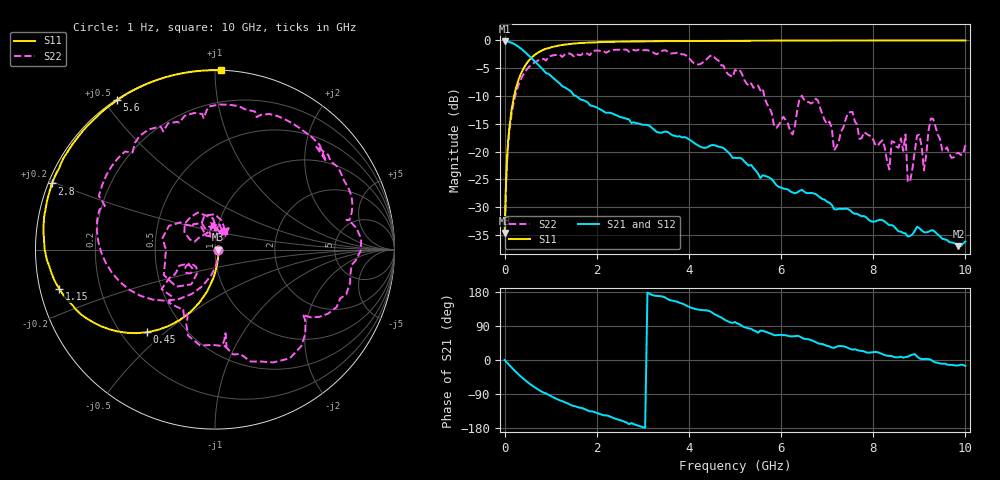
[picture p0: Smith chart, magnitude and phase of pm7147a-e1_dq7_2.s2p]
# GHz S DB R 50
! S-Parameters data
! Freq  dbS11  angS11  dbS21  angS21  dbS12  angS12  dbS22  angS22
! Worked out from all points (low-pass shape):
!   279 points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, 1 Hz to 10 GHz, reference 50 ohm
!   highest |S21| = -0.16 dB at 158.5 Hz (marker M1); lowest = -37.0 dB at 9.85 GHz (marker M2)
!   |S21| within 3 dB of the highest: start of sweep to 580.1 MHz
!   lowest |S11| = -34.6 dB at 100 Hz (marker M3), VSWR 1.04, Z = 51.9 - j1.4e-05 ohm
!   |S11| at or under -10 dB: start of sweep to 206.4 MHz
!   |S22| runs from -34.6 to -1.6 dB; largest |S21 - S12| = 0
!   S11 on the Smith chart (normalised r, x): 1 Hz: 1.04, -0.00; 450 MHz: 0.30, -0.44; 1.15 GHz: 0.06, -0.12; 2.8 GHz: 0.01, +0.20; 5.6 GHz: 0.00, +0.54; 10 GHz: 0.00, +1.03
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1e-09  -34.62 -0.0  -0.16 -0.0  -0.16 -0.0  -34.62 -0.0
1e-07  -34.62 -0.0  -0.16 -0.0  -0.16 -0.0  -34.62 -0.0
1.585e-07  -34.62 -0.0  -0.16 -0.0  -0.16 -0.0  -34.62 -0.0
0.15  -12.55 -100.5  -0.42 -19.5  -0.42 -19.5  -13.35 -108.9
0.45  -4.48 -129.5  -2.14 -53.9  -2.14 -53.9  -5.57 -154.8
1.15  -0.96 -165.9  -7.41 -103.8  -7.41 -103.8  -2.58 136.9
1.7  -0.44 178.6  -10.73 -127.8  -10.73 -127.8  -2.33 102.7
2.8  -0.18 157.9  -14.72 -169.0  -14.72 -169.0  -1.70 39.9
3.35  -0.13 149.9  -16.57 168.8  -16.57 168.8  -2.21 11.1
4.55  -0.09 134.6  -18.84 121.5  -18.84 121.5  -3.01 -62.8
5.05  -0.06 129.0  -21.14 96.3  -21.14 96.3  -5.50 -91.7
5.6  -0.05 123.2  -24.26 77.1  -24.26 77.1  -8.63 -143.5
6.25  -0.02 116.7  -27.34 62.5  -27.34 62.5  -16.93 -136.8
6.7  -0.02 112.6  -27.50 50.2  -27.50 50.2  -11.08 176.8
8.35  -0.01 99.1  -33.25 10.6  -33.25 10.6  -23.22 99.3
8.7  -0.00 96.6  -34.72 7.8  -34.72 7.8  -16.91 57.4
8.8  -0.00 95.9  -35.17 11.9  -35.17 11.9  -25.33 85.1
9  -0.00 94.5  -33.77 4.5  -33.77 4.5  -16.95 79.6
9.1  -0.00 93.9  -34.48 2.4  -34.48 2.4  -23.36 84.6
9.25  -0.00 92.9  -34.19 0.7  -34.19 0.7  -14.06 107.1
9.85  -0.00 89.0  -37.01 -14.2  -37.01 -14.2  -20.23 70.8
10  -0.00 88.1  -36.16 -15.7  -36.16 -15.7  -18.79 63.6
